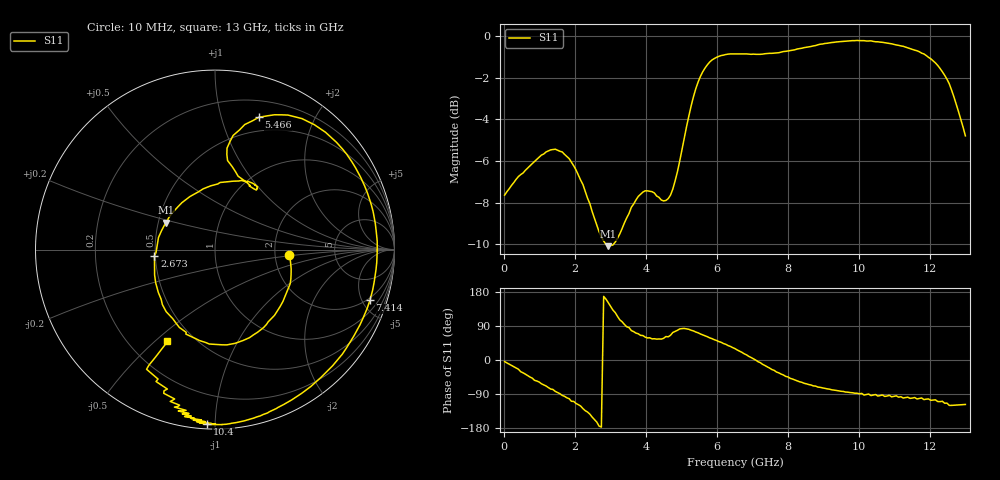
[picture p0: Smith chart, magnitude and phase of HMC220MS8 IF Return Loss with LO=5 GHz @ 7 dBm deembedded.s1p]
!Hittite Microwave Corporation
!12 Elizabeth Drive
!Chelmsford, MA 01824
!Tel: 978-250-3343
!Fax: 978-250-3373
!Device: HMC220MS8, 5-12 GHz, GaAS MMIC SMT Double-Balanced Mixer in 8-lead MSOP package
!Misc: IF Return Loss, LO = 5 GHz @ 7dBm, Room
# MHZ S MA R 50
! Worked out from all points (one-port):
!   201 points, 10 MHz to 13 GHz, reference 50 ohm
!   lowest |S11| = -10.1 dB at 2.933 GHz (marker M1), VSWR 1.91, Z = 27.4 + j9.14 ohm
!   |S11| at or under -10 dB: 2.865 GHz to 3.079 GHz (213.4 MHz wide, 7.18 % of centre)
!   S11 on the Smith chart (normalised r, x): 10 MHz: 2.40, -0.18; 2.673 GHz: 0.49, -0.04; 5.466 GHz: 0.36, +1.32; 7.414 GHz: 1.79, -5.74; 10.4 GHz: 0.03, -0.96; 13 GHz: 0.36, -0.55
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10  0.415 -4.3
789.4  0.494 -47.8
1244.05  0.53 -72.8
1633.75  0.527 -93.5
2153.35  0.451 -121.5
2672.95  0.339 -174.4
2932.75  0.313 151.3
3257.5  0.335 105.9
4036.9  0.425 58.2
4491.55  0.402 57.1
4881.25  0.472 78.3
5141.05  0.607 82.1
5465.8  0.776 71.7
5985.4  0.889 51.5
6505  0.906 30.0
7024.6  0.905 3.0
7414.3  0.908 -18.1
8128.75  0.925 -50.3
8843.2  0.953 -71.5
9752.5  0.974 -86.0
10402  0.971 -92.5
10921.6  0.958 -97.3
11051.5  0.952 -94.5
11246.35  0.945 -100.3
11376.25  0.937 -98.1
12155.65  0.862 -105.1
12545.35  0.768 -119.8
13000  0.576 -117.4
